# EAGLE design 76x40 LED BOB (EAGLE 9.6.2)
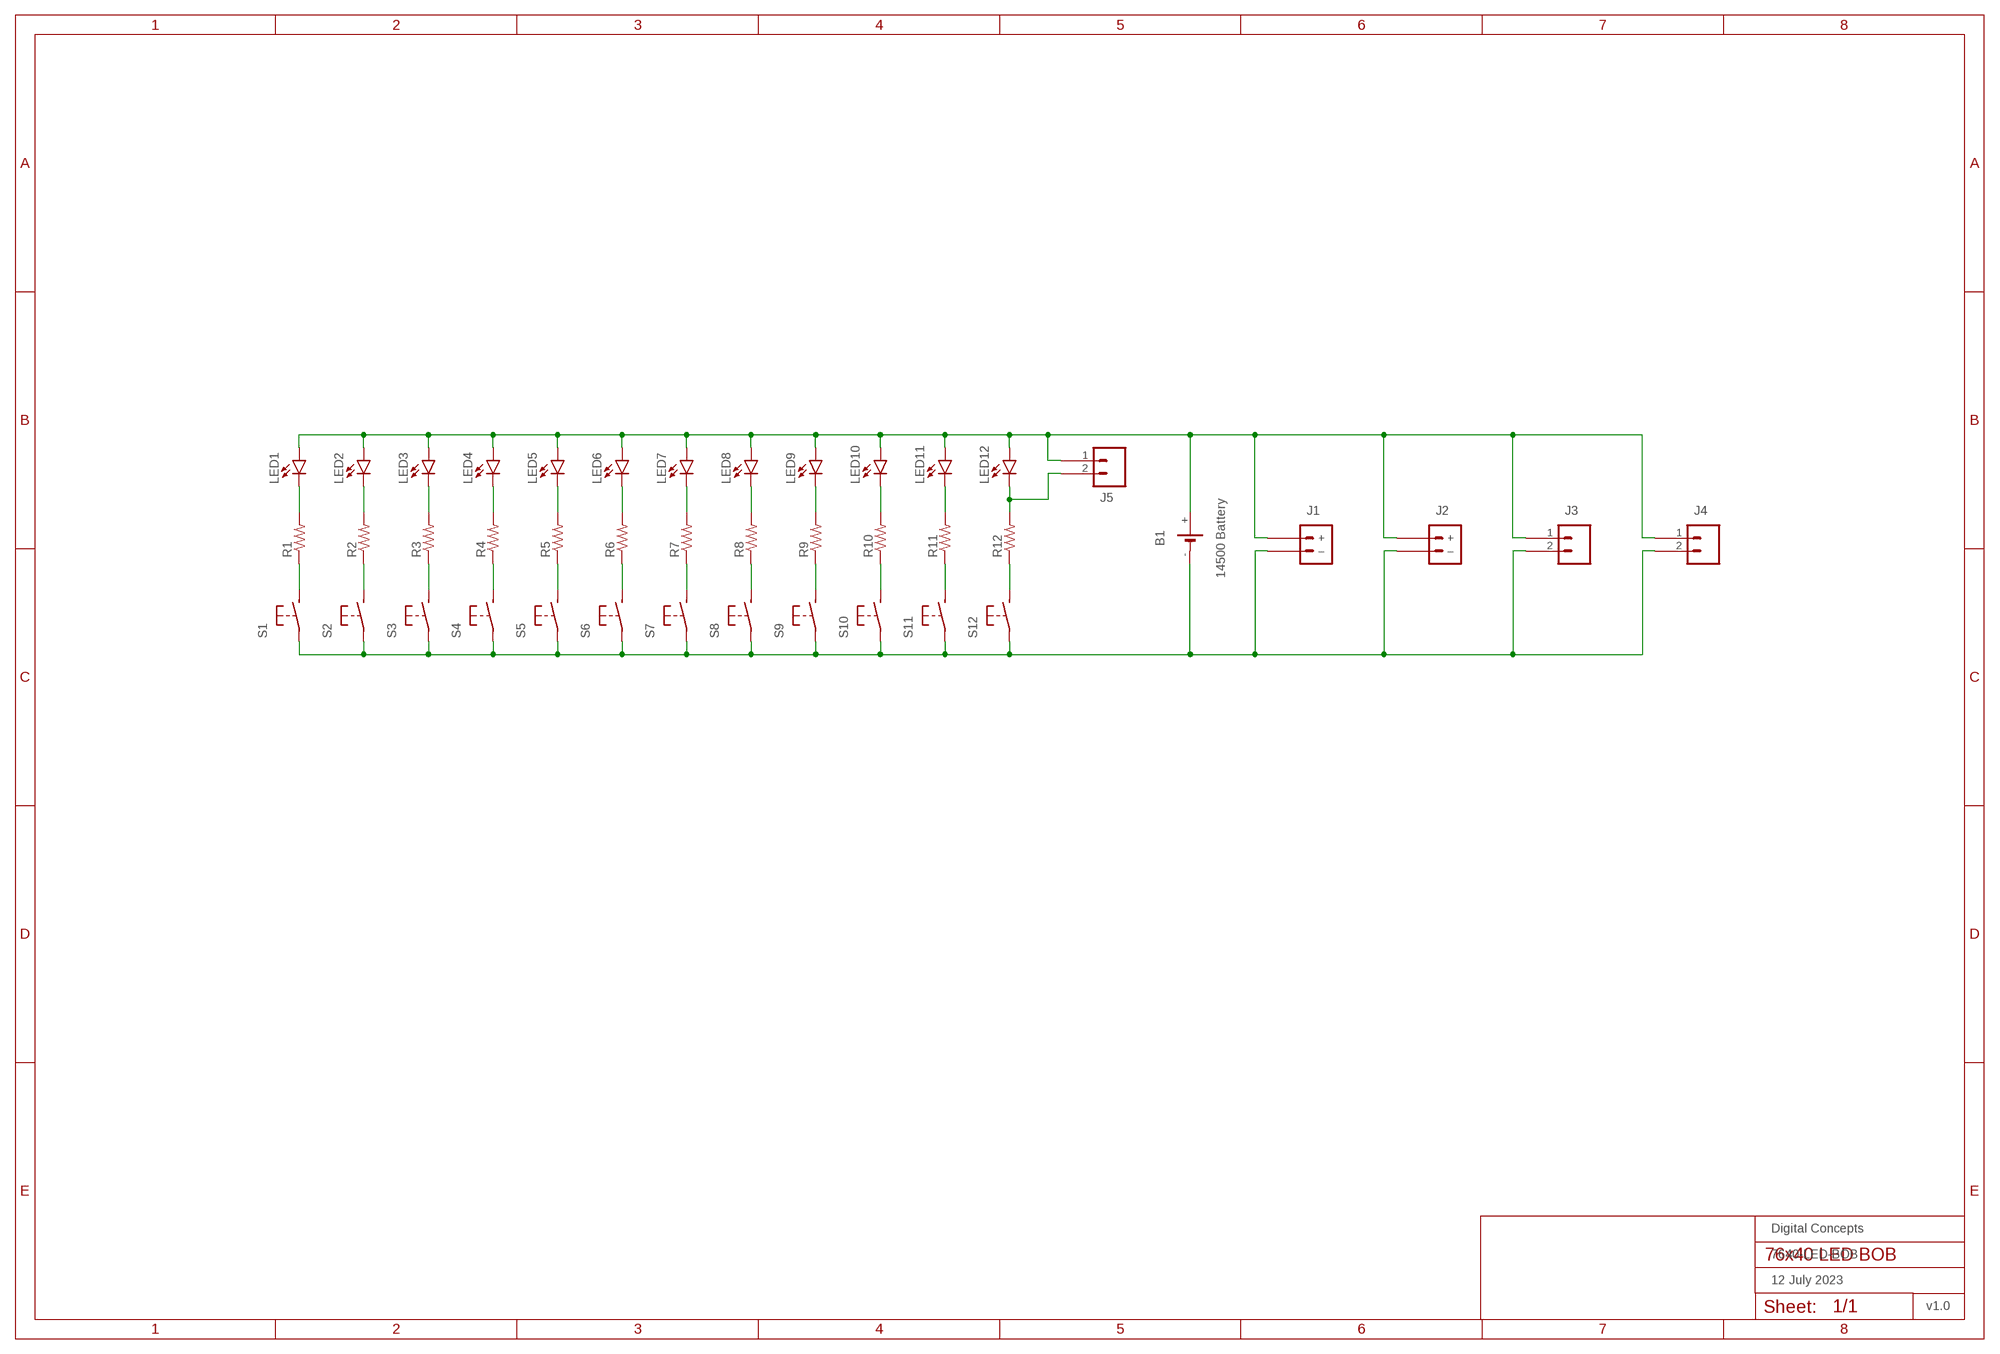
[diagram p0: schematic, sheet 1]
FRAME1 (FRAME-A3L-LOC): DATE: 12 July 2023; OWNER: Digital Concepts; TITLE: 7640-LED-BOB; VERSION: v1.0

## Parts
B1  14500 Battery  BATTERY-HOLDER-14500(AA)  [BATTERY-14500]
J1  JST-PH2.0-2-H-POWER  [JST-PH2.0-2-HORIZONTAL-POWER]
J2  JST-GH1.25-2-HORIZONTAL-POWER  [JST-GH1.25-2-HORIZONTAL]
J3  HEADER-1X2-GENERIC  [CONN_02-GENERIC]
J4  HEADER-1X2-GENERIC  [CONN_02-GENERIC]
J5  HEADER-1X2-GENERIC  [CONN_02-GENERIC]
LED1  LEDCHIP-LED0805  [CHIP-LED0805]
LED2  LEDCHIP-LED0805  [CHIP-LED0805]
LED3  LEDCHIP-LED0805  [CHIP-LED0805]
LED4  LEDCHIP-LED0805  [CHIP-LED0805]
LED5  LEDCHIP-LED0805  [CHIP-LED0805]
LED6  LEDCHIP-LED0805  [CHIP-LED0805]
LED7  LEDCHIP-LED0805  [CHIP-LED0805]
LED8  LEDCHIP-LED0805  [CHIP-LED0805]
LED9  LEDCHIP-LED0805  [CHIP-LED0805]
LED10  LEDCHIP-LED0805  [CHIP-LED0805]
LED11  LEDCHIP-LED0805  [CHIP-LED0805]
LED12  LEDCHIP-LED0805  [CHIP-LED0805]
R1  RESISTORR0805  [R0805]
R2  RESISTORR0805  [R0805]
R3  RESISTORR0805  [R0805]
R4  RESISTORR0805  [R0805]
R5  RESISTORR0805  [R0805]
R6  RESISTORR0805  [R0805]
R7  RESISTORR0805  [R0805]
R8  RESISTORR0805  [R0805]
R9  RESISTORR0805  [R0805]
R10  RESISTORR0805  [R0805]
R11  RESISTORR0805  [R0805]
R12  RESISTORR0805  [R0805]
S1  SWITCH-MOMENTARY-2-PIN  [SWITCH-2-PAD]
S2  SWITCH-MOMENTARY-2-PIN  [SWITCH-2-PAD]
S3  SWITCH-MOMENTARY-2-PIN  [SWITCH-2-PAD]
S4  SWITCH-MOMENTARY-2-PIN  [SWITCH-2-PAD]
S5  SWITCH-MOMENTARY-2-PIN  [SWITCH-2-PAD]
S6  SWITCH-MOMENTARY-2-PIN  [SWITCH-2-PAD]
S7  SWITCH-MOMENTARY-2-PIN  [SWITCH-2-PAD]
S8  SWITCH-MOMENTARY-2-PIN  [SWITCH-2-PAD]
S9  SWITCH-MOMENTARY-2-PIN  [SWITCH-2-PAD]
S10  SWITCH-MOMENTARY-2-PIN  [SWITCH-2-PAD]
S11  SWITCH-MOMENTARY-2-PIN  [SWITCH-2-PAD]
S12  SWITCH-MOMENTARY-2-PIN  [SWITCH-2-PAD]

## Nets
N$1: LED1.C R1.2
N$2: R1.1 S1.P$2(S)
N$4: J5.2 LED12.C R12.2
N$5: LED2.C R2.2
N$6: R2.1 S2.P$2(S)
N$9: LED3.C R3.2
N$10: R3.1 S3.P$2(S)
N$13: LED4.C R4.2
N$14: R4.1 S4.P$2(S)
N$17: LED5.C R5.2
N$18: R5.1 S5.P$2(S)
N$21: LED6.C R6.2
N$22: R6.1 S6.P$2(S)
N$25: LED7.C R7.2
N$26: R7.1 S7.P$2(S)
N$29: LED8.C R8.2
N$30: R8.1 S8.P$2(S)
N$33: LED9.C R9.2
N$34: R9.1 S9.P$2(S)
N$37: LED10.C R10.2
N$38: R10.1 S10.P$2(S)
N$41: LED11.C R11.2
N$42: R11.1 S11.P$2(S)
N$46: R12.1 S12.P$2(S)
N$49: B1.+ J1.+ J2.+ J3.1 J4.1 J5.1 LED1.A LED2.A LED3.A LED4.A LED5.A LED6.A LED7.A LED8.A LED9.A LED10.A LED11.A LED12.A
N$50: B1.- J1.-(–) J2.-(–) J3.2 J4.2 S1.P$1(P) S2.P$1(P) S3.P$1(P) S4.P$1(P) S5.P$1(P) S6.P$1(P) S7.P$1(P) S8.P$1(P) S9.P$1(P) S10.P$1(P) S11.P$1(P) S12.P$1(P)

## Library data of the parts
B1 = digitalconcepts:BATTERY-HOLDER-14500(AA): 14500 (AA) battery holder
J1 = digitalconcepts:JST-PH2.0-2-H-POWER: JST PH2.0 2P Right Angle Connector with power pin labelling
J2 = digitalconcepts:JST-GH1.25-2-HORIZONTAL-POWER: JST GH1.25 2P PTH Connector (Power)
J3-J5 = digitalconcepts:HEADER-1X2-GENERIC: Single Row 2-Pin Header
LED1-LED12 = digitalconcepts:LED: LED
R1-R12 = digitalconcepts:RESISTOR: Resistor; SPICEPREFIX: R
S1-S12 = digitalconcepts:SWITCH-MOMENTARY-2-PIN: 2 Pin Momentary Switch

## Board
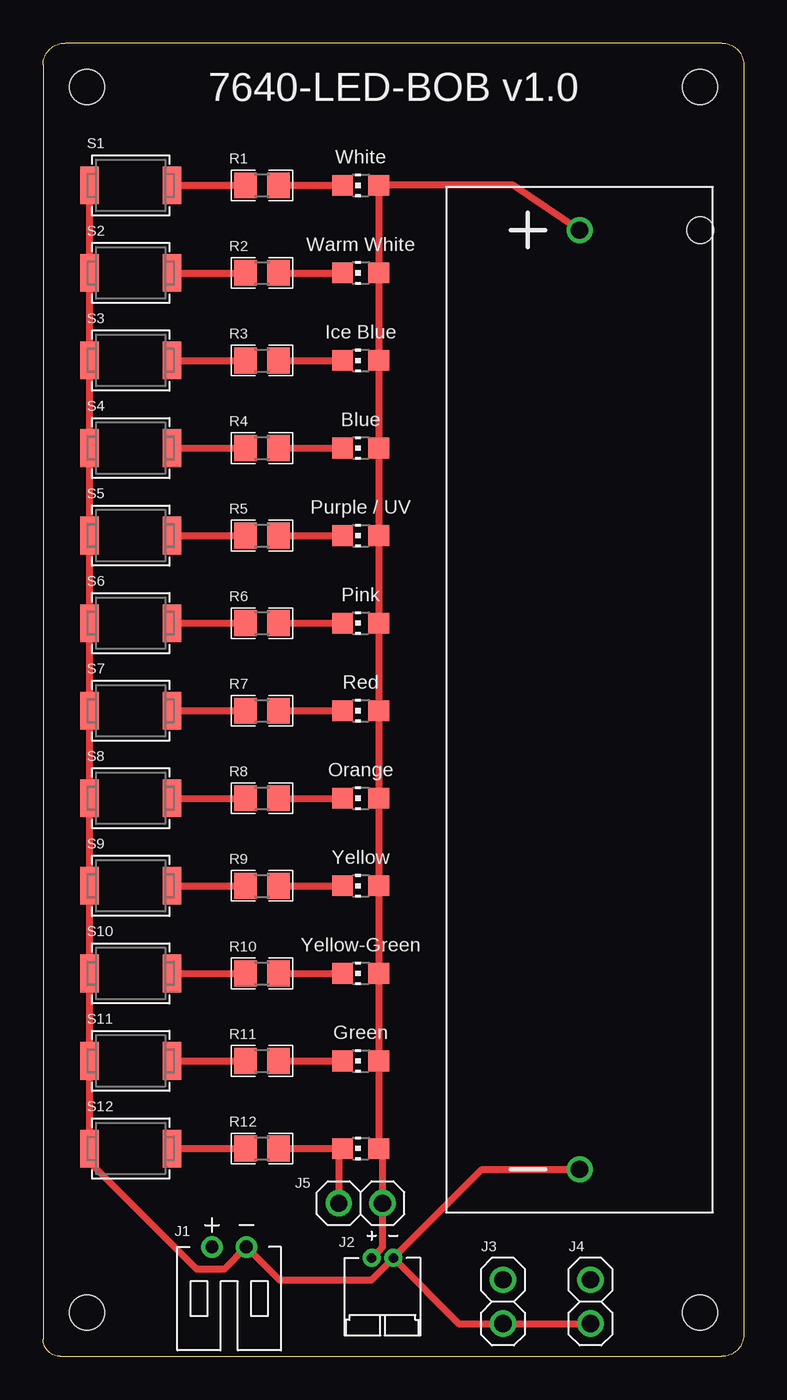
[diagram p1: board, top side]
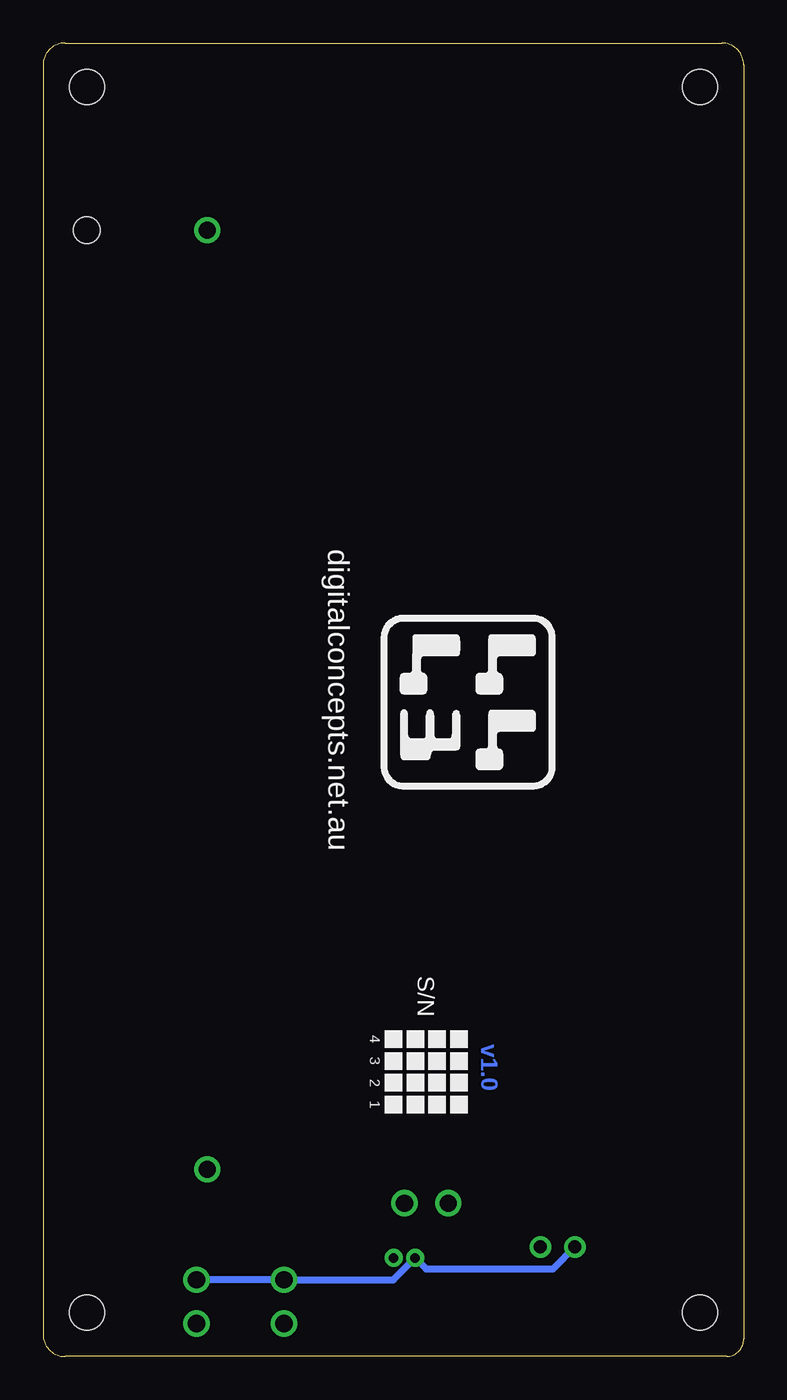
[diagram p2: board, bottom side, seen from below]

Size 40.64 x 76.2 mm. Coordinates in mm from the lower left corner, seen from the top.
Outline: 39.37,76.2 arc-90 40.64,74.93 40.64,1.27 arc-90 39.37,0 1,0 arc-90 0,1 0,74.93 arc-90 1.27,76.2 39.37,76.2
Copper layers (1*16): Top 0.035mm / dielectric 1.5mm / Bottom 0.035mm
Design rules "default *": minimum track width 6mil, minimum drill 0.35mm, track to track 6mil, track to pad 6mil, pad to pad 6mil, via to via 6mil, smd to smd 6mil, copper to edge 6mil, drill to drill 6mil, minimum pad ring 10mil, minimum via ring 8mil, stop-mask expansion 4mil, vias tented up to drill 0mil, thermal gap 0mil
Holes 2.03 mm at 2.54,73.66 2.54,2.54 38.1,2.54 38.1,73.66

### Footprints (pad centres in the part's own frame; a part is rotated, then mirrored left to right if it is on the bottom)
BATTERY-14500 = drill 1: + -27.25,0; - 27.25,0 | hole 1.524: -27.25,7
JST-PH2.0-2-HORIZONTAL-POWER = drill 0.75: + 1,0; - -1,0
JST-GH1.25-2-HORIZONTAL = drill 0.55 pad 1.016: + -0.625,0; - 0.625,0
CONN_02-GENERIC = drill 1 pad 1.524: 1 0,0; 2 2.54,0
CHIP-LED0805 = smd 1.2 x 1.2: A 0,-1.05; C 0,1.05
R0805 = smd 1.3 x 1.5: 1 -0.95,0; 2 0.95,0
SWITCH-2-PAD = smd 1.067 x 2.184: P$1 -2.4,0; P$2 2.4,0

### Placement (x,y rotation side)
B1  31.11,38.1 270 top
J1  10.79,6.35 180 top
J2  19.68,5.71 0 top
J3  26.67,4.45 270 top
J4  31.75,4.45 270 top
J5  19.68,8.89 180 top
LED1  18.41,67.94 90 top
LED2  18.41,62.87 90 top
LED3  18.41,57.78 90 top
LED4  18.41,52.7 90 top
LED5  18.41,47.62 90 top
LED6  18.41,42.55 90 top
LED7  18.41,37.47 90 top
LED8  18.41,32.38 90 top
LED9  18.41,27.3 90 top
LED10  18.41,22.23 90 top
LED11  18.41,17.14 90 top
LED12  18.41,12.06 90 top
R1  12.7,67.94 0 top
R2  12.7,62.87 0 top
R3  12.7,57.78 0 top
R4  12.7,52.7 0 top
R5  12.7,47.62 0 top
R6  12.7,42.55 0 top
R7  12.7,37.47 0 top
R8  12.7,32.38 0 top
R9  12.7,27.3 0 top
R10  12.7,22.23 0 top
R11  12.7,17.14 0 top
R12  12.7,12.06 0 top
S1  5.08,67.94 0 top
S2  5.08,62.87 0 top
S3  5.08,57.78 0 top
S4  5.08,52.7 0 top
S5  5.08,47.62 0 top
S6  5.08,42.55 0 top
S7  5.08,37.47 0 top
S8  5.08,32.38 0 top
S9  5.08,27.3 0 top
S10  5.08,22.23 0 top
S11  5.08,17.14 0 top
S12  5.08,12.06 0 top

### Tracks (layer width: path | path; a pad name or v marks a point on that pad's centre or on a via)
N$1
  Top 0.406: R1.2 LED1.C
N$2
  Top 0.406: S1.P$2 R1.1
N$4
  Top 0.406: R12.2 LED12.C 17.14,11.85 J5.2
N$5
  Top 0.406: R2.2 LED2.C
N$6
  Top 0.406: S2.P$2 R2.1
N$9
  Top 0.406: R3.2 LED3.C
N$10
  Top 0.406: S3.P$2 R3.1
N$13
  Top 0.406: R4.2 LED4.C
N$14
  Top 0.406: S4.P$2 R4.1
N$17
  Top 0.406: R5.2 LED5.C
N$18
  Top 0.406: S5.P$2 R5.1
N$21
  Top 0.406: R6.2 LED6.C
N$22
  Top 0.406: S6.P$2 R6.1
N$25
  Top 0.406: R7.2 LED7.C
N$26
  Top 0.406: S7.P$2 R7.1
N$29
  Top 0.406: R8.2 LED8.C
N$30
  Top 0.406: S8.P$2 R8.1
N$33
  Top 0.406: R9.2 LED9.C
N$34
  Top 0.406: S9.P$2 R9.1
N$37
  Top 0.406: R10.2 LED10.C
N$38
  Top 0.406: S10.P$2 R10.1
N$41
  Top 0.406: R11.2 LED11.C
N$42
  Top 0.406: S11.P$2 R11.1
N$46
  Top 0.406: S12.P$2 R12.1
N$49
  Top 0.406: B1.+ 27.28,67.94 LED1.A LED2.A LED3.A LED4.A LED5.A LED6.A LED7.A LED8.A LED9.A LED10.A LED11.A LED12.A 19.68,11.85 J5.1 19.68,6.34 19.43,6.08 J2.+
  Bottom 0.406: J1.+ 11.06,5.08 18.43,5.08 J2.+ 20.33,4.45 J3.1 J4.1
N$50
  Top 0.406: S1.P$1 S2.P$1 S3.P$1 S4.P$1 S5.P$1 S6.P$1 S7.P$1 S8.P$1 S9.P$1 S10.P$1 S11.P$1 S12.P$1 2.68,11.29 8.89,5.08 10.53,5.08 J1.- 13.7,4.45 19.05,4.45 J2.- | J2.- 25.45,10.85 B1.- | J2.- 24.12,1.91 J3.2 J4.2

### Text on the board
Bottom: v1.0
tPlace: 7640-LED-BOB v1.0 | White | Warm White | Ice Blue | Blue | Purple / UV | Pink | Red | Orange | Yellow | Yellow-Green | Green
bPlace: digitalconcepts.net.au | S/N | 4 | 3 | 2 | 1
